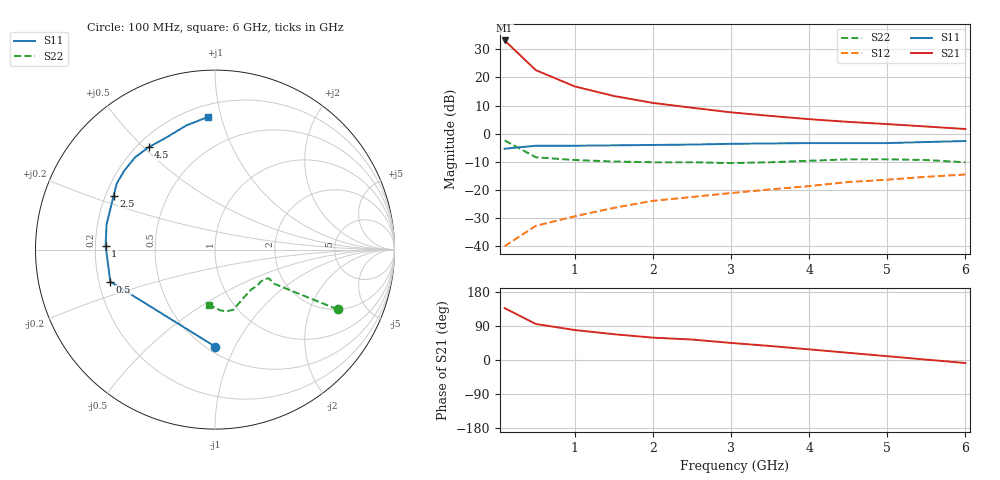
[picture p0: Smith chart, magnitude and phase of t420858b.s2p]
!AT-42085
!S-PARAMETERS at Vce=8V Ic=35mA. LAST UPDATED 07-21-92
# ghz s ma r 50
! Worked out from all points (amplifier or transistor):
!   13 points, 100 MHz to 6 GHz, reference 50 ohm
!   highest |S21| = 33.1 dB at 100 MHz (marker M1)
!   |S21| within 3 dB of that: start of sweep to 213.6 MHz
!   unconditionally stable (mu >= 1): 842.5 MHz to 4.25 GHz
!   at 1 GHz: K = 1.10, MAG = 21.2 dB, |S12| = -29.4 dB
!   at 3 GHz: K = 1.14, MAG = 12.1 dB, |S12| = -21.1 dB
!   at 6 GHz: K = 0.84, MSG = 8.1 dB, |S12| = -14.5 dB
!   S11 on the Smith chart (normalised r, x): 100 MHz: 0.55, -0.84; 500 MHz: 0.25, -0.14; 1 GHz: 0.24, +0.02; 2.5 GHz: 0.23, +0.24; 4.5 GHz: 0.24, +0.52; 6 GHz: 0.28, +0.91
0.1  0.54 -90.0  45.38 137.0  0.01 66.0  0.76 -26.0
0.5  0.61 -163.0  13.45 95.0  0.023 52.0  0.38 -30.0
1  0.61 178.0  6.9 79.0  0.034 61.0  0.34 -28.0
1.5  0.62 167.0  4.67 68.0  0.048 68.0  0.32 -31.0
2  0.63 156.0  3.52 59.0  0.064 66.0  0.31 -36.0
2.5  0.64 152.0  2.89 54.0  0.075 68.0  0.31 -40.0
3  0.66 146.0  2.39 45.0  0.088 69.0  0.3 -48.0
3.5  0.67 139.0  2.07 37.0  0.102 67.0  0.31 -58.0
4  0.68 131.0  1.81 28.0  0.117 65.0  0.33 -67.0
4.5  0.68 123.0  1.62 19.0  0.138 60.0  0.35 -73.0
5  0.68 114.0  1.48 10.0  0.152 56.0  0.35 -79.0
5.5  0.71 103.0  1.34 1.0  0.171 50.0  0.34 -85.0
6  0.74 93.0  1.21 -8.0  0.188 46.0  0.31 -96.0
